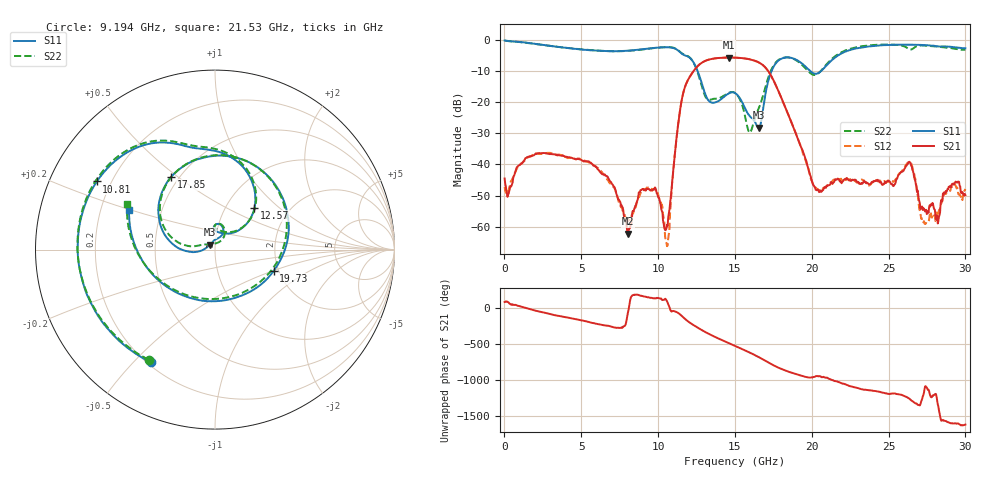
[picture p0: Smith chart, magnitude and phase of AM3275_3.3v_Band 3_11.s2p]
!Keysight Technologies,N5245B,MY58422270,A.16.20.02
!Date: Thursday, March 27, 2025 02:03:07
!Correction: S11(C  2-Port  )
!S21(C  2-Port  )
!S12(C  2-Port  )
!S22(C  2-Port  )
!S2P File: Measurements: S11, S21, S12, S22:
# Hz S  dB  R 50
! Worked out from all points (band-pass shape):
!   801 points, 10 MHz to 30 GHz, reference 50 ohm
!   highest |S21| = -5.61 dB at 14.63 GHz (marker M1); lowest = -62.3 dB at 8.032 GHz (marker M2)
!   |S21| within 3 dB of the highest: 12.53 GHz to 16.94 GHz (4.41 GHz wide, 29.9 % of centre)
!   lowest |S11| = -28.2 dB at 16.54 GHz (marker M3), VSWR 1.08, Z = 47.3 + j2.68 ohm
!   |S11| at or under -10 dB: 12.58 GHz to 17.38 GHz (4.804 GHz wide, 32.1 % of centre); 19.92 GHz to 20.6 GHz (681.6 MHz wide, 3.36 % of centre)
!   |S22| runs from -29.8 to -0.2 dB; largest |S21 - S12| = 0.0085
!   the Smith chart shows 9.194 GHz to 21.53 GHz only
!   S11 on the Smith chart (normalised r, x): 9.194 GHz: 0.21, -0.56; 10.81 GHz: 0.15, +0.26; 12.57 GHz: 1.36, +0.70; 17.85 GHz: 0.45, +0.47; 19.73 GHz: 1.88, -0.51; 21.53 GHz: 0.32, +0.20
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1e7  -0.12 -3.1  -44.51 76.4  -47.32 -34.0  -0.18 -4.6
1.322062e9  -0.77 -82.7  -38.47 -1.8  -38.78 -3.1  -0.80 -83.2
2.7091e9  -1.70 -158.8  -36.49 -76.7  -36.35 -77.2  -1.71 -159.6
5.033325e9  -3.04 92.3  -38.66 -177.4  -38.36 -178.4  -2.99 91.0
8.032325e9  -3.42 -55.6  -62.31 -74.1  -57.65 135.6  -3.48 -57.9
9.194438e9  -2.83 -119.5  -48.43 149.7  -47.87 147.3  -2.89 -121.1
1.001916e10  -2.41 -164.8  -50.69 131.4  -49.94 120.1  -2.42 -165.7
1.08064e10  -2.38 150.1  -51.49 -38.5  -53.61 -41.2  -2.30 149.6
1.155615e10  -4.43 106.1  -18.79 -119.1  -18.83 -119.3  -4.30 105.5
1.256831e10  -9.90 46.5  -8.42 82.8  -8.42 82.7  -10.36 44.5
1.343052e10  -20.02 66.9  -6.13 -18.1  -6.12 -18.2  -19.16 74.6
1.463012e10  -17.09 88.2  -5.61 -135.3  -5.61 -135.4  -16.88 86.8
1.5005e10  -17.05 76.3  -5.64 -170.3  -5.64 -170.4  -16.98 73.4
1.654199e10  -28.19 133.5  -7.16 35.4  -7.16 35.4  -22.05 160.4
1.785405e10  -6.49 121.1  -16.66 -113.8  -16.65 -113.5  -6.33 117.4
1.972842e10  -9.18 -20.1  -40.60 116.7  -40.99 115.3  -9.78 -25.8
2.002832e10  -10.43 -54.4  -45.67 113.4  -45.64 113.3  -11.02 -62.7
2.152782e10  -5.57 155.3  -44.75 63.7  -44.97 72.5  -5.16 152.6
2.501416e10  -1.58 38.8  -45.32 -115.2  -45.44 -107.2  -1.41 36.0
2.64012e10  -1.49 4.6  -39.43 171.2  -39.56 169.7  -3.04 3.1
2.733839e10  -1.61 -20.2  -54.71 -49.4  -59.05 50.6  -1.77 -19.3
3e10  -2.63 -112.9  -49.89 -178.3  -47.88 -179.5  -3.09 -113.0
